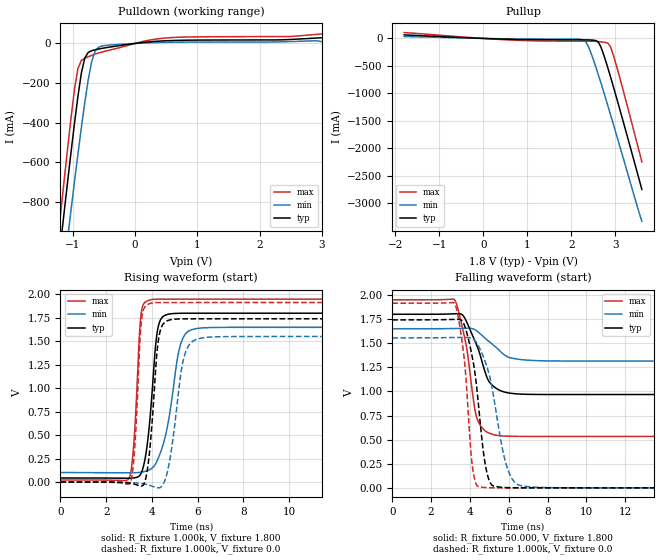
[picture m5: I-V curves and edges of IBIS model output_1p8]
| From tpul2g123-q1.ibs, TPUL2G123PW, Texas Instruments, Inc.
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|   Output Models
|   Model output_1p8
[Model] output_1p8
Model_type Output
Polarity   Non-Inverting
Enable   Active-High
Vmeas = 1.8v
Cref = 15pf
C_comp   2.293pF   1.969pF   2.650pF
[Temperature Range]   27.000   0.125k   -40.000
[Voltage Range]   1.800V   1.650V   1.950V
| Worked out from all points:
|   slope of the pulldown table from 0 to 0.27 V, typ, clamps not added: 30.2 ohm
|   slope of the pullup table from 0 to 0.27 V, typ, clamps not added: 35.1 ohm
|   rising waveform, R_fixture 1.000k, V_fixture 1.800: 20-80 % time 365ps typ, 628ps min, 245ps max; typ from 0.044 V to 1.8 V
|   rising waveform, R_fixture 1.000k, V_fixture 0.0: 20-80 % time 319ps typ, 494ps min, 230ps max; typ from 0 V to 1.74 V
|   falling waveform, R_fixture 50.000, V_fixture 1.800: 20-80 % time 882ps typ, 1.15ns min, 650ps max; typ from 1.8 V to 0.968 V
|   falling waveform, R_fixture 1.000k, V_fixture 0.0: 20-80 % time 627ps typ, 885ps min, 461ps max; typ from 1.74 V to 0 V
[Pulldown]
|Voltage   I(typ)   I(min)   I(max)
-1.8V     -2.76A     -2.941A    -2.715A
-1.25V    -1.16A     -1.426A    -1.018A
-1.195V   -1.004A    -1.277A    -852.3mA
-1.14V    -849.5mA   -1.13A     -689.3mA
-1.085V   -697.3mA   -984.3mA   -529.6mA
-1.03V    -548.5mA   -840.3mA   -375.7mA
-920mV    -269.2mA   -560.5mA   -127.1mA
-810mV    -74.72mA   -300.5mA   -75.1mA
-700mV    -36.92mA   -93.98mA   -60.5mA
-590mV    -28.42mA   -19.95mA   -48.53mA
510mV     13.64mA    5.429mA    27.77mA
3.6V      35.75mA    7.114mA    65.96mA
[Pullup]
|Voltage   I(typ)   I(min)   I(max)
-1.8V     64mA       34.95mA    106.7mA
575mV     -14.92mA   -7.919mA   -27.15mA
2.28V     -26.03mA   -31.3mA    -50.38mA
2.335V    -26.35mA   -74.03mA   -50.51mA
2.39V     -27.16mA   -157.6mA   -50.66mA
2.61V     -67.19mA   -658mA     -57.12mA
2.72V     -265.6mA   -941.2mA   -67.23mA
2.83V     -543.4mA   -1.232A    -86.63mA
2.885V    -691.6mA   -1.38A     -147.7mA
2.995V    -996.9mA   -1.678A    -419.1mA
3.105V    -1.309A    -1.979A    -734.7mA
3.6V      -2.749A    -3.328A    -2.247A
[Ramp]
| variable   typ   min   max
dV/dt_r   1.045/0.319n   0.933/0.494n   1.149/0.230n
dV/dt_f   1.054/0.655n   0.929/0.970n   1.157/0.474n
R_load = 1.000k
[Rising Waveform]
R_fixture= 1.000k
V_fixture= 1.800
V_fixture_min= 1.650
V_fixture_max= 1.950
|time   V(typ)   V(min)   V(max)
0s        43.74mV    102.1mV    21.87mV
3.01ns    41.53mV    98.88mV    43.6mV
3.218ns   45.06mV    99.44mV    441.2mV
3.521ns   89.27mV    105.2mV    1.776V
3.98ns    862mV      143.8mV    1.945V
4.187ns   1.514V     206.5mV    1.949V
4.367ns   1.725V     308.9mV    1.95V
5.238ns   1.799V     1.453V     1.95V
5.898ns   1.8V       1.635V     1.95V
50ns      1.8V       1.65V      1.95V
[Rising Waveform]
R_fixture= 1.000k
V_fixture= 0.0
V_fixture_min= 0.0
V_fixture_max= 0.0
|time   V(typ)   V(min)   V(max)
0s        520.3nV    409.2nV    764.2nV
3.062ns   -13.2mV    -4.591mV   -2.097mV
3.259ns   -23.38mV   -8.466mV   401.7mV
3.552ns   -41.95mV   -16.64mV   1.736V
4.035ns   725.4mV    -45.56mV   1.91V
4.243ns   1.431V     -60.48mV   1.913V
4.453ns   1.67V      -38.72mV   1.914V
5.409ns   1.74V      1.334V     1.914V
6.149ns   1.74V      1.534V     1.914V
50ns      1.742V     1.555V     1.915V
[Falling Waveform]
R_fixture= 50.000
V_fixture= 1.800
V_fixture_min= 1.650
V_fixture_max= 1.950
|time   V(typ)   V(min)   V(max)
0s        1.8V       1.65V      1.95V
3.225ns   1.805V     1.652V     1.945V
3.81ns    1.73V      1.655V     1.474V
4.181ns   1.558V     1.647V     911.1mV
4.355ns   1.477V     1.627V     724.9mV
4.916ns   1.128V     1.528V     574.2mV
5.425ns   1.023V     1.442V     543.6mV
6.055ns   982.2mV    1.35V      535.2mV
7.921ns   968mV      1.317V     533.3mV
50ns      967.8mV    1.314V     533.3mV
[Falling Waveform]
R_fixture= 1.000k
V_fixture= 0.0
V_fixture_min= 0.0
V_fixture_max= 0.0
|time   V(typ)   V(min)   V(max)
0s        1.742V     1.555V     1.915V
3.224ns   1.747V     1.559V     1.906V
3.822ns   1.619V     1.559V     1.062V
4.106ns   1.372V     1.55V      256.7mV
4.422ns   898.8mV    1.478V     13.97mV
4.753ns   289.2mV    1.326V     3.91mV
5.059ns   48.46mV    1.119V     1.244mV
5.898ns   2.848mV    223.5mV    61.03uV
6.728ns   278.6uV    19.01mV    31.41uV
50ns      1.498uV    6.944uV    240.2nV
